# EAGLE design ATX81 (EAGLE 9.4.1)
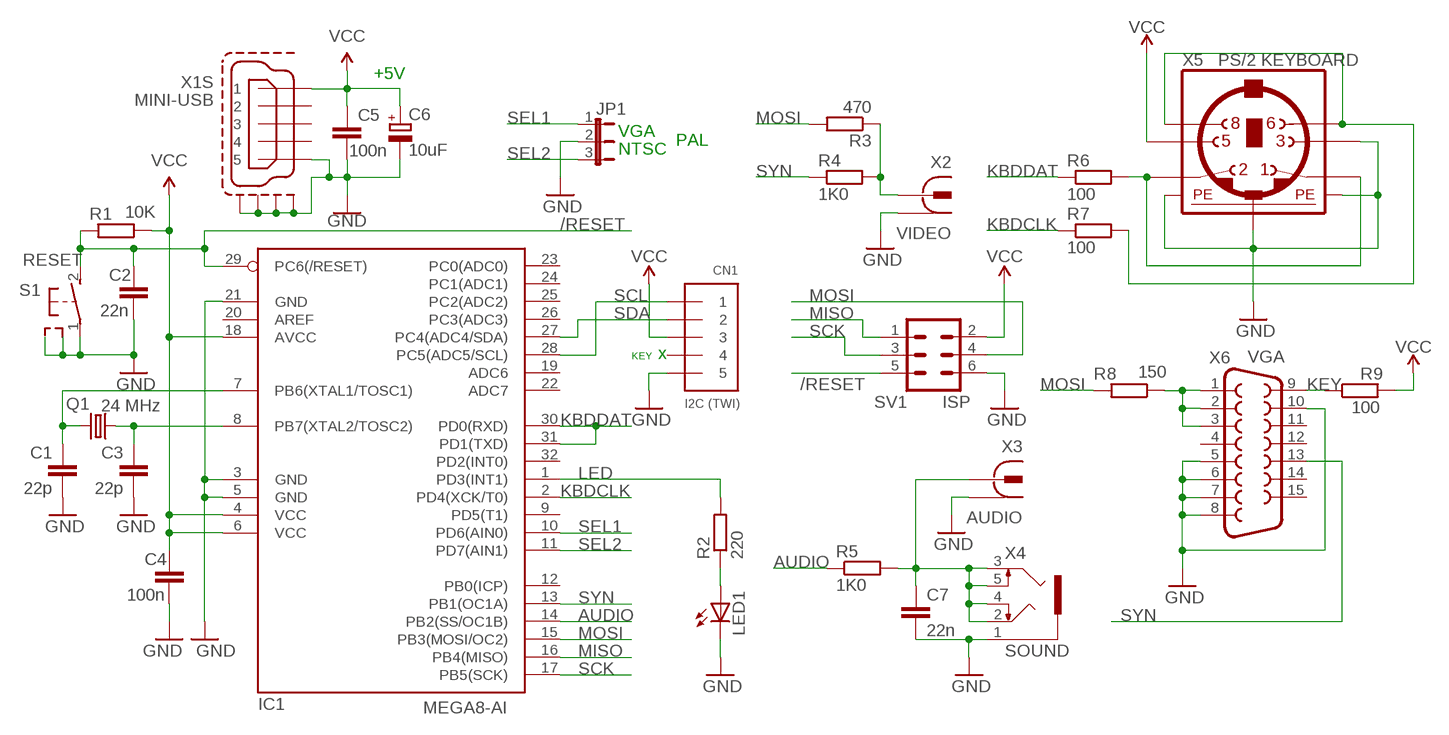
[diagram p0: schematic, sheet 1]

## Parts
C1  22p  C-EU050-024X044  [C050-024X044]
C2  22n  C-EU050-024X044  [C050-024X044]
C3  22p  C-EU050-024X044  [C050-024X044]
C4  100n  C-EU050-024X044  [C050-024X044]
C5  100n  C-EU050-024X044  [C050-024X044]
C6  10uF  CPOL-EUE2.5-5  [E2,5-5]
C7  22n  C-EU050-024X044  [C050-024X044]
CN1  I2C (TWI)  1X51X05-BIG2  [1X05-BIG]
IC1  MEGA8-AI  [TQFP32-08]
JP1  JP2E  [JP2]
LED1  LED3MM  [LED3MM]
Q1  24 MHz  CRYSTALHC49U-V  [HC49U-V]
R1  10K  R-EU_0204/7  [0204/7]
R2  220  R-EU_0204/7  [0204/7]
R3  470  R-EU_0204/7  [0204/7]
R4  1K0  R-EU_0204/7  [0204/7]
R5  1K0  R-EU_0204/7  [0204/7]
R6  100  R-EU_0204/7  [0204/7]
R7  100  R-EU_0204/7  [0204/7]
R8  150  R-EU_0204/7  [0204/7]
R9  100  R-EU_0204/7  [0204/7]
S1  RESET  31-XX  [B3F-31XX]
SV1  ISP  ML6L  [ML6L]
X1  MINI-USB  MINI-USB-SHIELD-UX60-MB-5ST  [UX60-MB-5ST]
X2  VIDEO  736880-49  [736880-49]
X3  AUDIO  736880-49  [736880-49]
X4  SOUND  1503_09  [1503_09]
X5  PS/2 KEYBOARD  MINI_DIN_6  [M_DIN6]
X6  VGA  F15HDH  [HDF15H]

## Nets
/RESET: C2.1 IC1.29(PC6(/RESET)) R1.2 S1.2(S) SV1.5
AUDIO: IC1.14(PB2(SS/OC1B)) R5.1
GND: C1.1 C2.2 C3.1 C4.2 C5.2 C6.- C7.2 CN1.5 IC1.3(GND) IC1.5(GND) IC1.21(GND) JP1.2 LED1.K(C) S1.1(P) S1.3 S1.4 SV1.6 X1.5 X1.M1(S:S1) X1.M2(S:S2) X1.M3(S:S3) X1.M4(S:S4) X2.1 X2.1@1 X2.1@2 X3.1 X3.1@1 X3.1@2 X4.1 X5.3 X5.SH1(PE1) X5.SH2(PE2) X5.SH3(PE3) X6.5 X6.6 X6.7 X6.8 X6.10
KBDCLK: IC1.2(PD4(XCK/T0)) R7.1
KBDDAT: IC1.30(PD0(RXD)) IC1.31(PD1(TXD)) R6.1
KEY: R9.1 X6.9
LED: IC1.1(PD3(INT1)) R2.2
MISO: IC1.16(PB4(MISO)) SV1.1
MOSI: IC1.15(PB3(MOSI/OC2)) R3.2 R8.2 SV1.4
N$1: C7.1 R5.2 X3.2 X4.2 X4.3 X4.4 X4.5
N$2: LED1.A R2.1
N$3: R6.2 X5.1 X5.2
N$4: R7.2 X5.6 X5.8
N$15: C1.2 IC1.7(PB6(XTAL1/TOSC1)) Q1.2
N$16: C3.2 IC1.8(PB7(XTAL2/TOSC2)) Q1.1
RGB_VIDEO: R8.1 X6.1 X6.2 X6.3
SCK: IC1.17(PB5(SCK)) SV1.3
SCL: CN1.1 IC1.28(PC5(ADC5/SCL))
SDA: CN1.2 IC1.27(PC4(ADC4/SDA))
SEL1: IC1.10(PD6(AIN0)) JP1.1
SEL2: IC1.11(PD7(AIN1)) JP1.3
SYN: IC1.13(PB1(OC1A)) R4.1 X6.13
VCC: C4.1 C5.1 C6.+ CN1.3 IC1.4(VCC) IC1.6(VCC) IC1.18(AVCC) R1.1 R9.2 SV1.2 X1.1 X5.5
VIDEO: R3.1 R4.2 X2.2
Unconnected: CN1.4 IC1.9(PD5(T1)) IC1.12(PB0(ICP)) IC1.19(ADC6) IC1.20(AREF) IC1.22(ADC7) IC1.23(PC0(ADC0)) IC1.24(PC1(ADC1)) IC1.25(PC2(ADC2)) IC1.26(PC3(ADC3)) IC1.32(PD2(INT0)) X1.2 X1.3 X1.4 X6.4 X6.11 X6.12 X6.14 X6.15

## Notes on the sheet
- +5V
- VGA
- PAL
- NTSC
- KEY | x

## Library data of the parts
C1-C5 C7 = rcl:C-EU: CAPACITOR, European symbol; SPICEPREFIX: C
C6 = rcl:CPOL-EU: POLARIZED CAPACITOR, European symbol; SPICEPREFIX: C
CN1 = adafruit:1X5
IC1 = atmel:MEGA8: MICROCONTROLLER 8 Kbytes FLASH, 1 kbytes SRAM, 512 bytes EEPROM, USART, 6-channel 10 bit ADC, 2-channel 8 bit ADC Pin compatible with Atmega48, ATMega88, ATMega168 Source: avr.lbr; MPN: ATMEGA8-16AU; OC_FARNELL: 9171371; OC_NEWARK: 73M8863
JP1 = jumper:JP2E: JUMPER
LED1 = adafruit:LED: LED
Q1 = crystal:CRYSTAL: CRYSTAL; OC_FARNELL: 1666969; OC_NEWARK: unknown
R1-R9 = rcl:R-EU_: RESISTOR, European symbol; SPICEPREFIX: R
S1 = switch-omron:31-XX: OMRON SWITCH; MPN: B3F-3100; OC_FARNELL: 959704; OC_NEWARK: 36M3582
SV1 = con-ml:ML6L: HARTING; OC_FARNELL: unknown; OC_NEWARK: unknown
X1 = con-hirose:MINI-USB-SHIELD-: MINI USB Connector Source: http://www.hirose.co.jp/cataloge_hp/e24000019.pdf; OC_FARNELL: unknown; OC_NEWARK: unknown
X2 X3 = con-conrad:736880-49: Cinch Connector ( RCA Jack )
X4 = con-lumberg:1503_09: Jack connectors according to JISC 6560, 3.5 mm Klinkeneinbaukupplung nach JISC 6560, 3,5 mm, 3-polig/ stereo, abgewinkelte Ausführung, mit 2 Öffnern und Lötaugen, für Leiterplatten Rückseitenmontage Source: http://www.lumberg.com/Produkte/PDFs/1503_09.pdf; OC_FARNELL: 1243244; OC_NEWARK: unknown
X5 = mini_din:MINI_DIN_6
X6 = adafruit:F15: SUB-D HDH is also known as a 'right angle VGA' connector

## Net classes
0 default: width 0.6 mm, drill 0.3 mm

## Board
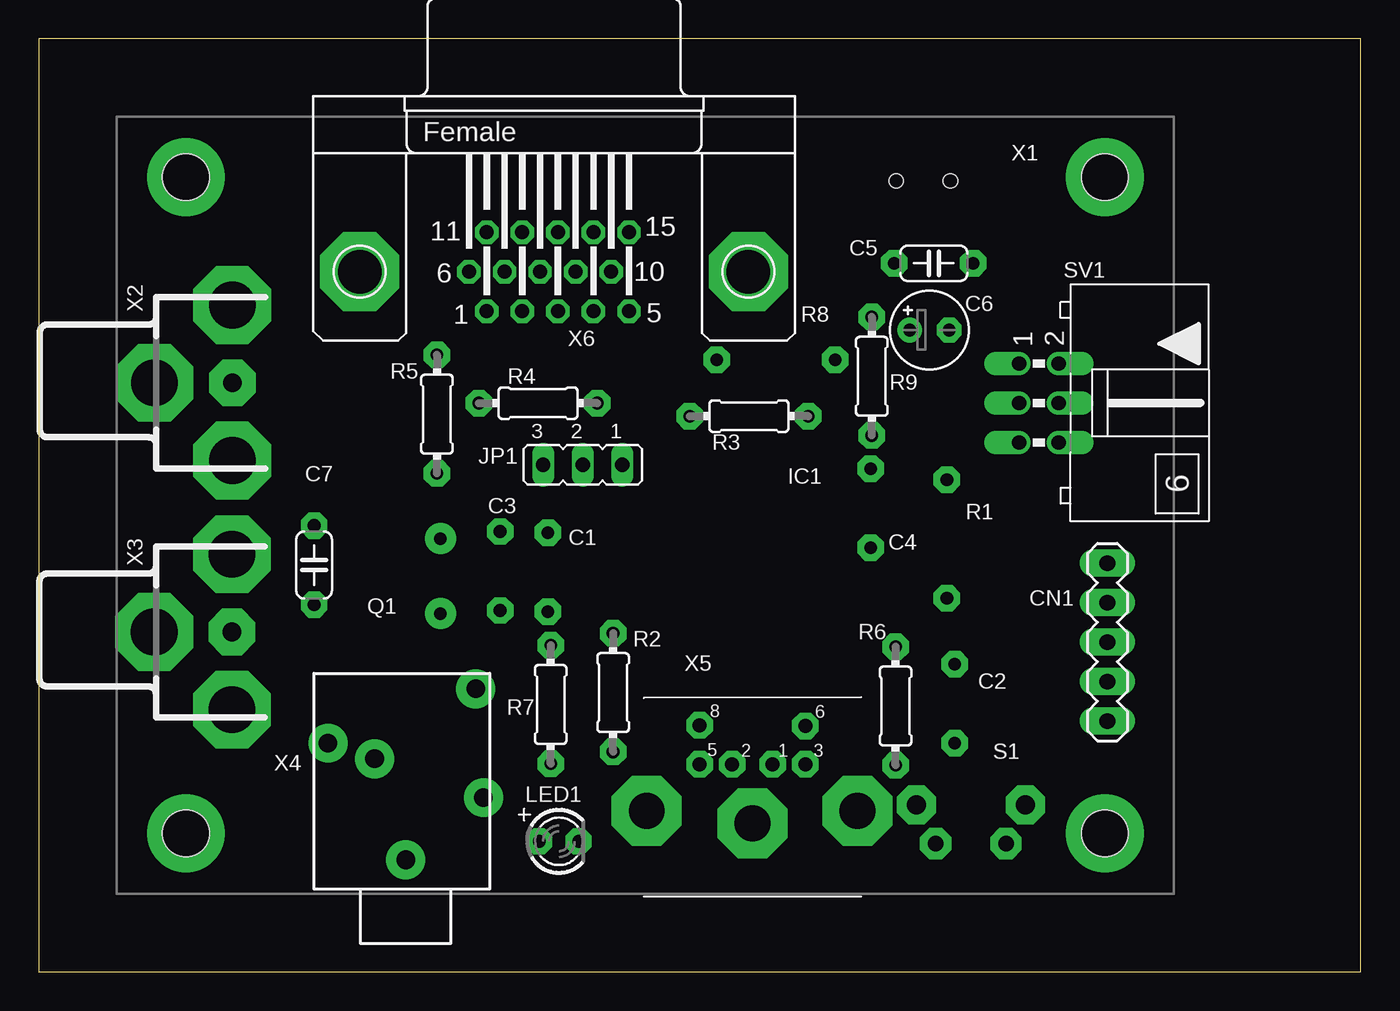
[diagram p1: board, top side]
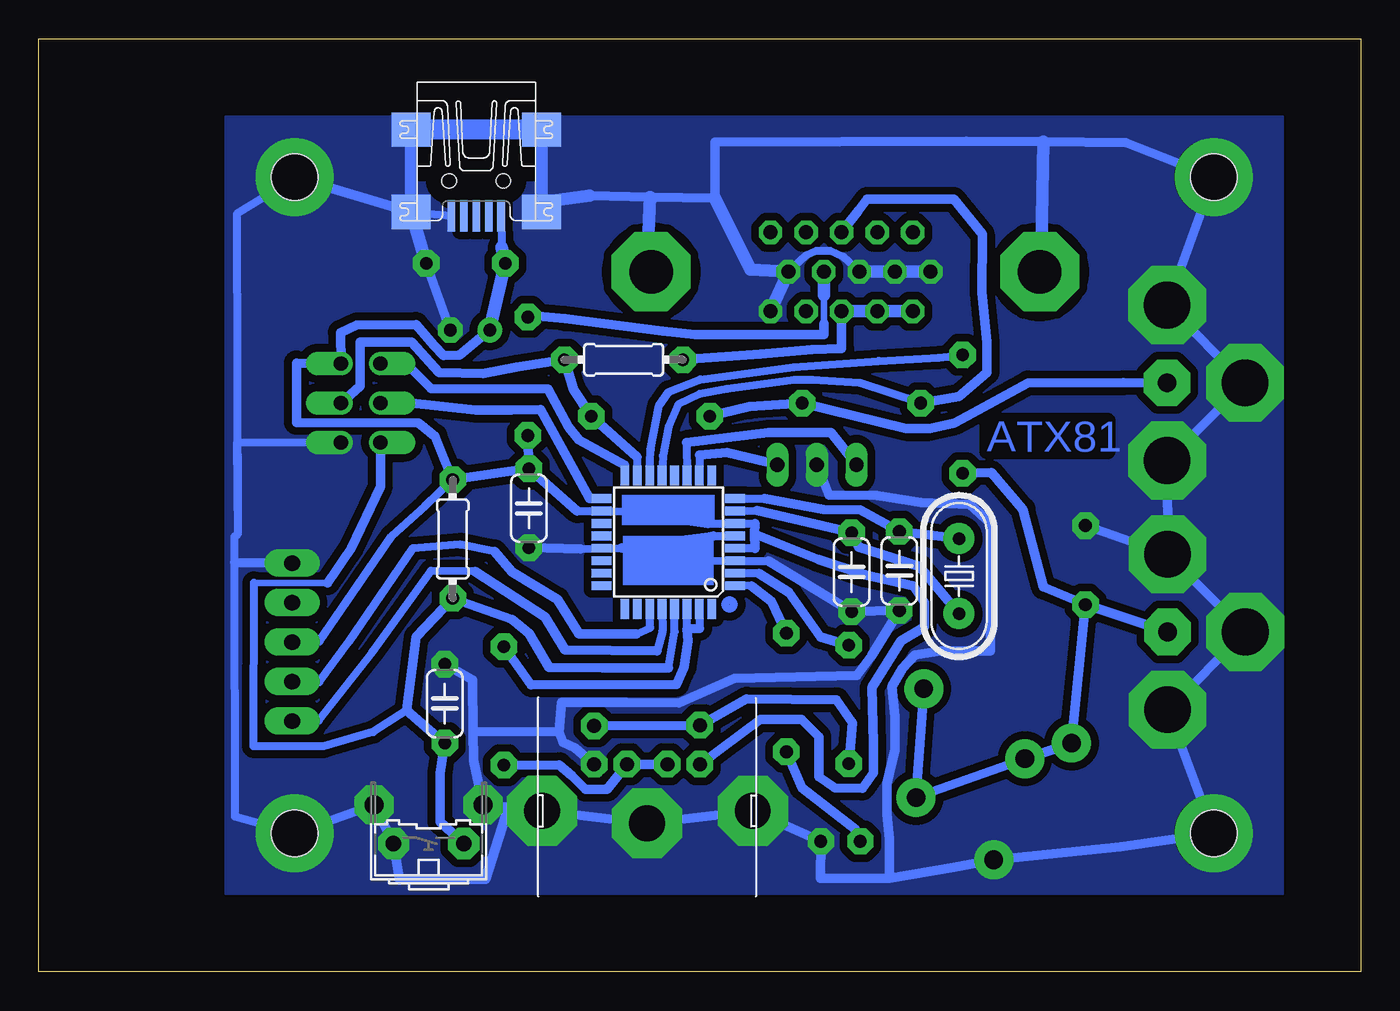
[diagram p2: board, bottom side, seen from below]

Size 85 x 60 mm. Coordinates in mm from the lower left corner, seen from the top.
Outline: 0,0 85,0 85,60 0,60 0,0
Copper layers (1*16): Top 0.035mm / dielectric 1.5mm / Bottom 0.035mm
Design rules "default": minimum track width 6mil, minimum drill 0.35mm, track to track 6mil, track to pad 6mil, pad to pad 6mil, via to via 6mil, smd to smd 6mil, copper to edge 40mil, drill to drill 6mil, minimum pad ring 10mil, minimum via ring 8mil, stop-mask expansion 4mil, vias tented up to drill 0mil, thermal gap 10mil
Holes 3 mm at 9.45,51.1 68.55,51.1 68.55,8.9 9.45,8.9

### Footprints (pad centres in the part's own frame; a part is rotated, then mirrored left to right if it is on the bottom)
C050-024X044 = drill 0.813 pad 1.7 octagon: 1 -2.54,0; 2 2.54,0
E2,5-5 = drill 0.813 pad 1.6: + -1.27,0 | drill 0.813 pad 1.6 octagon: - 1.27,0
1X05-BIG = drill 1.016 pad 1.778 long: 1 -5.08,0; 2 -2.54,0; 3 0,0; 4 2.54,0; 5 5.08,0
TQFP32-08 = smd 1.27 x 0.559: 1 -4.293,2.8; 2 -4.293,2; 3 -4.293,1.2; 4 -4.293,0.4; 5 -4.293,-0.4; 6 -4.293,-1.2; 7 -4.293,-2; 8 -4.293,-2.8; 17 4.293,-2.8; 18 4.293,-2; 19 4.293,-1.2; 20 4.293,-0.4; 21 4.293,0.4; 22 4.293,1.2; 23 4.293,2; 24 4.293,2.8 | smd 0.559 x 1.27: 9 -2.8,-4.293; 10 -2,-4.293; 11 -1.2,-4.293; 12 -0.4,-4.293; 13 0.4,-4.293; 14 1.2,-4.293; 15 2,-4.293; 16 2.8,-4.293; 25 2.8,4.293; 26 2,4.293; 27 1.2,4.293; 28 0.4,4.293; 29 -0.4,4.293; 30 -1.2,4.293; 31 -2,4.293; 32 -2.8,4.293
JP2 = drill 0.914 long: 1 -2.54,0; 2 0,0; 3 2.54,0
LED3MM = drill 0.813 pad 1.676 octagon: A -1.27,0; K 1.27,0
HC49U-V = drill 0.813 pad 2: 1 -2.413,0; 2 2.413,0
0204/7 = drill 0.813 pad 1.7 octagon: 1 -3.81,0; 2 3.81,0
B3F-31XX = drill 1 pad 2 octagon: 1 -2.261,-1.245; 2 2.261,-1.245 | drill 1.2 pad 2.5 octagon: 3 -3.505,1.245; 4 3.505,1.245
ML6L = drill 0.914 pad 1.5 offset: 1 -2.54,-1.27; 2 -2.54,1.27; 3 0,-1.27; 4 0,1.27; 5 2.54,-1.27; 6 2.54,1.27
UX60-MB-5ST = smd 2 x 0.5: 1 2.25,1.6; 2 2.25,0.8; 3 2.25,0; 4 2.25,-0.8; 5 2.25,-1.6 | smd 2.2 x 2.5: M1 -3.3,-4.2; M2 -3.3,4.2; M3 2,4.2; M4 2,-4.2 | hole 0.9: 0,-1.75; 0,1.75
736880-49 = drill 3 pad 5 octagon: 1 -2.5,0; 1@1 2.5,-5; 1@2 2.5,5 | drill 1.2 pad 3 octagon: 2 2.5,0
1503_09 = drill 1.2 pad 2.5: 1 0,-2; 2 -5,-6; 3 5,-9.5; 4 -4.5,-13; 5 2,-8.5
M_DIN6 = drill 0.9 pad 1.7 octagon: 1 -1.3,-3.75; 2 1.3,-3.75; 3 -3.4,-3.75; 5 3.4,-3.75; 6 -3.4,-6.2; 8 3.4,-6.25 | drill 2.3 pad 4.5 octagon: SH1 6.8,-0.75; SH2 0,0.05; SH3 -6.75,-0.75
HDF15H = drill 0.9 pad 1.5 octagon: 1 4.329,2.54; 2 2.043,2.54; 3 -0.243,2.54; 4 -2.529,2.54; 5 -4.815,2.54; 6 5.472,0; 7 3.186,0; 8 0.9,0; 9 -1.386,0; 10 -3.672,0; 11 4.329,-2.54; 12 2.043,-2.54; 13 -0.243,-2.54; 14 -2.529,-2.54; 15 -4.815,-2.54 | drill 2.8 pad 5.08 octagon: P$1 -12.5,0; P$2 12.5,0

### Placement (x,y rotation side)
C1  32.74,25.7 90 bottom
C2  58.9,17.24 90 bottom
C3  29.66,25.78 90 bottom
C4  53.49,29.82 270 bottom
C5  57.55,45.56 0 top
C6  57.27,41.27 0 top
C7  17.7,26.16 90 top
CN1  68.72,21.2 90 top
IC1  44.52,27.63 180 bottom
JP1  34.97,32.61 180 top
LED1  33.44,8.39 0 top
Q1  25.83,25.45 270 bottom
R1  58.39,27.83 270 bottom
R2  36.93,17.95 90 top
R3  45.67,35.73 0 top
R4  32.1,36.57 0 top
R5  25.6,35.86 270 top
R6  55.09,17.09 270 top
R7  32.91,17.19 270 top
R8  47.39,39.37 180 bottom
R9  53.56,38.3 270 top
S1  59.94,9.49 0 bottom
SV1  64.31,36.58 270 top
X1  56.87,50.87 270 bottom
X2  9.94,37.88 0 top
X3  9.91,21.85 0 top
X4  23.59,5.2 180 top
X5  45.89,9.6 180 top
X6  33.13,45.02 180 top

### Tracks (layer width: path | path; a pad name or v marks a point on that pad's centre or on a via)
/RESET
  Bottom 0.406: 71.17,25.02 66.44,25.02
  Bottom 0.508: 44.52,19.55 44.12,21.87 IC1.29 | 61.34,16.8 63.5,15.41 66.7,14.5 71.19,14.5 71.17,25.02
  Bottom 0.61: S1.2 59.2,9.65 59.2,12.77 C2.1 61.34,16.8 60.73,21.54 R1.2 54.58,22.65 53.49,21.76 52.19,19.58 48.74,19.55 44.52,19.55 | 66.44,25.02 64.92,27.23 63.04,31.21 SV1.5
AUDIO
  Bottom 0.508: IC1.14 45.66,33.58 45.11,36.42 44.52,37.28 42.47,38.1 36.47,38.88 30.98,39.29 27.12,39.49 R5.1
GND  (via drill 1 pad 5)
  Bottom 0.508: X1.M4 X1.5 | 47.52,27.25 IC1.21 50.16,27.2 | 41.6,28.01 IC1.5 | 41.93,26.44 IC1.3 38.1,26.41 | X6.8 33.25,45.97 34.11,46.35 35.02,46.35 35.66,46.07 X6.10 | v68.55,8.9 72.39,9.98 72.4,26.31 72.41,27.99 72.19,28.17 | 72.19,28.17 72.23,34.08 SV1.6 | 72.19,28.17 72.23,48.79 68.96,50.8 68.35,51.04
  Bottom 0.6: 30.45,10.15 30.45,12.11 29.94,14.27 29.94,16.41 30.15,18.36 29.47,19.5 28.67,20.37 27,20.65
  Bottom 0.61: 52.67,49.5 X1.M3 | X1.M4 68.35,51.04 v68.55,51.1 | C5.2 C6.- | 47.52,27.25 41.9,27.97 | 41.9,27.97 41.6,28.01 | 41.9,27.97 41.93,26.44 | 38.1,26.41 C1.1 C3.1 31.45,20.31 32.38,19.05 40.28,18.87 43.84,17.29 47.22,17.32 51.38,17.32 51.53,15.44 | 54.8,10.6 X5.SH3 X5.SH2 X5.SH1 LED1.K 34.74,6.02 30.3,6 | 54.8,10.6 S1.4 57.05,13.59 57.09,15.44 | 30.3,6 26.16,6.7 X4.1 15.44,8.05 v9.45,8.9 X3.1@1 X3.1 X3.1@2 | X3.1@2 X2.1@1 X2.1 X2.1@2 v9.45,51.1 15.11,53.34 20.42,53.38 25.34,53.41 41.52,53.36 41.52,49.76 45.69,49.83 49.58,49.91 | X3.1@2 C7.2 | 27,20.65 23.82,20.65 23.82,28.27 23.82,28.41 23.82,28.85 25.12,30.04 28.27,30.17 31.11,30.63 34.19,30.65 JP1.2 | 30.45,10.15 30.3,8.5 30.3,6 | v68.55,8.9 S1.3 S1.1 61.79,5.89 56.26,5.94 54.8,10.6 | C4.2 50.16,27.2 | C2.2 57.09,18.77 57.09,15.44 | X5.3 50.52,14.4 51.3,14.75 51.53,15.44 | 51.53,15.44 57.09,15.44 | CN1.5 72.4,26.31
  Bottom 0.813: X1.M1 X1.M4 C5.2 | X1.M2 52.67,49.5 49.58,49.91 | X6.6 X6.7 X6.8 | X6.5 X6.10 39.24,45.16 41.52,49.76 | 20.42,53.38 20.55,46.76 | 45.69,49.83 45.82,46.83
  Bottom 1.27: X1.M2 X1.M1
  pour Bottom (isolate 0.5, no thermals): 73,55 5,55 5,5 73,5
KBDCLK
  Bottom 0.508: 38.68,25.62 IC1.2
  Bottom 0.61: R7.1 34.74,21.54 36.75,24.41 38.68,25.62
KBDDAT
  Bottom 0.508: 43.32,22.05 IC1.30 | IC1.31 42.52,22.09
  Bottom 0.61: 42.52,22.09 43.32,22.05 43.25,21.28 43.51,19.58 43.99,18.49 53.34,18.46 R6.1
KEY
  Bottom 0.406: 34.52,43.51 34.52,41.7
  Bottom 0.61: 34.52,41.7 34.52,40.99 42.82,40.97 44.9,41.2 51.15,42.01 53.28,42.21 R9.1
  Bottom 0.813: X6.9 34.52,43.51
LED
  Bottom 0.508: 39.16,24.81 IC1.1
  Bottom 0.61: R2.2 37.89,23.82 39.16,24.81
MISO
  Bottom 0.508: 47.34,32.58 IC1.16
  Bottom 0.61: SV1.1 61.34,39.09 59.79,37.51 52.27,37.49 50.92,35.05 50.26,34.19 47.34,32.58
MOSI
  Bottom 0.508: 46.53,33.09 IC1.15
  Bottom 0.61: 46.53,33.09 R3.2 50.61,37.46 R8.2 54.28,38.88 56.44,38.48 59.25,38.55 61.03,40.51 62,40.51 64.33,40.48 64.33,37.66 SV1.4
N$1
  Bottom 0.61: X4.4 X4.2 X4.5 X4.3 C7.1 | C7.1 20.39,24.74 21.71,29.74 23.75,32.1 R5.2 | C7.1 X3.2
N$2
  Bottom 0.61: LED1.A 32.48,9.17 35.94,11.83 R2.1
N$3
  Bottom 0.61: X5.2 X5.1 48.46,11.73 49.86,11.73 50.72,12.59 51.53,13.31 R6.2
N$4
  Bottom 0.61: X5.6 X5.8 39.49,17.55 33.7,17.5 32.69,16 R7.2
N$15
  Bottom 0.508: IC1.7 38.81,29.66
  Bottom 0.61: 38.81,29.66 C1.2 32.3,27.33 28.37,26.08 Q1.2
N$16
  Bottom 0.508: IC1.8 38.35,30.43
  Bottom 0.61: 38.35,30.43 34.54,29.74 32.15,29.71 C3.2 Q1.1
RGB_VIDEO
  Bottom 0.61: R8.1 38.58,39.72 35.28,40 33.37,40.08 X6.3
  Bottom 0.813: X6.3 X6.2 X6.1
SCK
  Bottom 0.61: SV1.3 61.31,36.6 56.92,36.11 54.61,36.14 52.73,36.17 51.38,33.73 49.6,30.45 IC1.17
SCL
  Bottom 0.508: IC1.28 44.9,21.89 45.26,20.62 | 56.94,25.75 59.79,25.78 63.55,20.57 67,16.15 CN1.1
  Bottom 0.61: 45.26,20.62 51.15,20.7 52.45,22.83 56.94,25.75
SDA
  Bottom 0.508: 46.55,21.71 45.69,22.12 IC1.27 | 55.7,27.02 57.91,27.48 60.96,27.23 65.1,21.2 66.98,18.64 CN1.2
  Bottom 0.61: 55.7,27.02 54.55,25.7 51.66,23.95 50.26,21.71 46.55,21.71
SEL1
  Bottom 0.508: 42.52,33.22 IC1.10
  Bottom 0.61: JP1.1 40.74,33.4 42.52,33.22
SEL2
  Bottom 0.508: 43.35,34.03 IC1.11
  Bottom 0.61: JP1.3 34.06,34.67 38.1,34.69 43.35,34.03
SYN
  Bottom 0.508: R4.1 32.2,37.87 35.28,38.07 36.39,38.07 40.74,37.49 42.49,37.16 43.89,36.47 44.5,35.07 44.88,33.19 IC1.13
  Bottom 0.61: X6.13 32.28,48.97 31.75,49.68 26.16,49.68 24.33,47.44 24.36,43.68 24.05,40.48 24.02,38.55 25.83,37 R4.1
VCC
  Bottom 0.508: X1.1 55.24,46.6 | 50.39,29.64 IC1.18 47.37,29.61 | 41.98,28.82 IC1.6 38.96,28.82 | 38.96,27.23 IC1.4 | CN1.3 66.98,21.23 62.3,28.01 60.14,29.99 R1.1
  Bottom 0.6: 34.87,26.51 31.85,25.52 28.75,24.81 28.06,23.75 28.06,22.17 29.56,21.28 31.42,18.28 31.34,14.7 31.34,12.8 32.05,11.81 33.8,11.83 34.84,12.54 34.84,15.11
  Bottom 0.61: C4.1 R1.1 58.95,32.97 59.51,34.44 60.58,35.3 68.42,35.33 68.42,39.16 SV1.2 65.6,41.12 64.56,41.6 60.75,41.63 59.59,40.28 58.98,39.65 57.93,39.67 C6.+ | C4.1 50.39,29.64 | 47.37,29.61 41.98,28.82 | 38.96,28.82 38.97,28.15 | 38.97,28.15 38.96,27.23 | X5.5 38.6,16.23 35.96,16.23 34.84,15.11 | 38.97,28.15 34.87,26.51 | C4.1 R9.2
  Bottom 0.813: 55.24,46.6 C5.1 C6.+
VIDEO
  Bottom 0.61: X2.2 15.27,37.89 21.38,37.87 25.3,35.73 26.13,35.3 27.68,34.95 29.25,34.94 R4.2 39.29,36.34 R3.1
(copper drawn outside any net)
  shapes: Bottom area x2, Bottom circle x1

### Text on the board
Bottom: ATX81
tValues: NTSC | VGA | PAL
